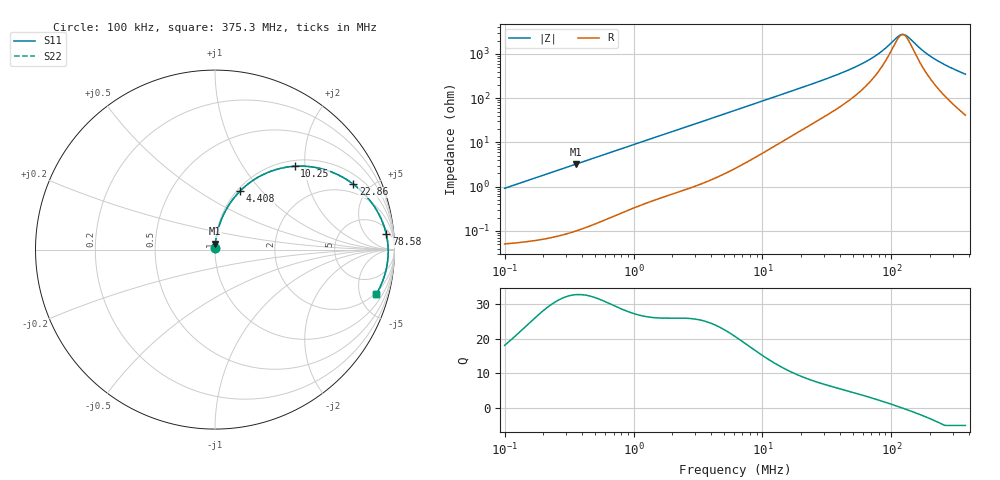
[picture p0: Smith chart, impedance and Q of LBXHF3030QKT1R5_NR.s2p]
! LBXHF3030QKT1R5_NR  S-PARAMETER MODEL  ( General Type )
! Model Generated by TAIYO YUDEN Corporation (http://www.ty-top.com)
! Version 1.0
! TAIYO YUDEN Control No. 210113NI43SB-FBB
! Copyright(c) 2021 TAIYO YUDEN CO.,LTD. All Rights Reserved.
! Product Description (link to TY-COMPAS)
! https://ds.yuden.co.jp/TYCOMPAS/or/detail?pn=LBXHF3030QKT1R5MNR&u=M
! Products Name : Inductors
! Characteristics :
!  Inductance : 1.5 uH , SRF(min) : 80 MHz , DC Resistance(max) : 0.046 Ohm
!  Rated Current : Saturation :1800 mA , Temp Rise : 1600 mA
!  Case Size : 3.0 x 3.0 / 0.118 x 0.118 [mm/inch] , Thickness : 1.5 / 0.059 [mm/inch]
!  (Conditions: Temperature = 25 degC , DC Bias Current/Voltage = 0A / 0V)
! External Node Assignments :
!  1  o---GGG---o  2
! GND o---------o GND
! Frequency Range : 0.1MHz  -  375.343504MHz  [ 402 STEP ]
# MHz S RI R 50
! Freq[MHz].  S11 Real  S11 Imag  S21 Real  S21 Imag  S12 Real  S12 Imag  S22 Real  S22 Imag
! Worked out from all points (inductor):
!   401 points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, 100 kHz to 375.3 MHz, reference 50 ohm
!   read as one part in series: L = 1.46 uH near 104.2 kHz
!   highest Q = 32.7 at 358.1 kHz (marker M1), where L = 1.45 uH
!   self-resonance near 122.2 MHz
!   S11 on the Smith chart (normalised r, x): 100 kHz: 1.00, +0.02; 4.408 MHz: 1.03, +0.77; 10.25 MHz: 1.12, +1.77; 22.86 MHz: 1.47, +3.92; 78.58 MHz: 9, +18; 375.3 MHz: 1.83, -6.93
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0.1  0.000592 0.00917  0.9994 -0.00917  0.9994 -0.00917  0.000592 0.00917
0.358127  0.00205 0.0325  0.9979 -0.0325  0.9979 -0.0325  0.00205 0.0325
0.396933  0.0024 0.036  0.9976 -0.036  0.9976 -0.036  0.0024 0.036
1.575555  0.0241 0.1353  0.9759 -0.1353  0.9759 -0.1353  0.0241 0.1353
2.803133  0.0645 0.2271  0.9355 -0.2271  0.9355 -0.2271  0.0645 0.2271
4.407956  0.1384 0.3249  0.8616 -0.3249  0.8616 -0.3249  0.1384 0.3249
6.253894  0.2382 0.4022  0.7618 -0.4022  0.7618 -0.4022  0.2382 0.4022
10.24746  0.4436 0.4644  0.5564 -0.4644  0.5564 -0.4644  0.4436 0.4644
14.84108  0.6117 0.4453  0.3883 -0.4453  0.3883 -0.4453  0.6117 0.4453
22.86247  0.7702 0.3648  0.2298 -0.3648  0.2298 -0.3648  0.7702 0.3648
24.31819  0.7881 0.3506  0.2119 -0.3506  0.2119 -0.3506  0.7881 0.3506
48.95057  0.9189 0.1857  0.0811 -0.1857  0.0811 -0.1857  0.9189 0.1857
63.96269  0.9427 0.1277  0.0573 -0.1277  0.0573 -0.1277  0.9427 0.1277
78.57555  0.9545 0.0857  0.0455 -0.0857  0.0455 -0.0857  0.9545 0.0857
96.52685  0.9616 0.0453  0.0384 -0.0453  0.0384 -0.0453  0.9616 0.0453
113.7985  0.9645 0.0137  0.0355 -0.0137  0.0355 -0.0137  0.9645 0.0137
126.1296  0.9652 -0.00607  0.0348 0.00607  0.0348 0.00607  0.9652 -0.00607
136.9498  0.965 -0.0219  0.035 0.0219  0.035 0.0219  0.965 -0.0219
178.9494  0.9604 -0.075  0.0396 0.075  0.0396 0.075  0.9604 -0.075
210.9691  0.954 -0.1094  0.046 0.1094  0.046 0.1094  0.954 -0.1094
281.3999  0.9343 -0.1748  0.0657 0.1748  0.0657 0.1748  0.9343 -0.1748
375.3435  0.8991 -0.2474  0.1009 0.2474  0.1009 0.2474  0.8991 -0.2474
